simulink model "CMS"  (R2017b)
settings: Solver=FixedStepDiscrete  StartTime=0.0  StopTime=10.0  FixedStep=0.01  RelTol=1e-3  EnableMultiTasking=on
undefined symbols (not defined in the file): ASWTYPE_FALSE, ASWTYPE_TRUE, CcCMS_CANSendDelay_ms, CcCMS_ChrgMaxPackVoltLimt_V, CcCMS_PeakVoltCh_V, CcCMS_PeakVoltDisCh_V, CcSOC_DispSOCHighThrhd_pct, CMS09D_RUNTIME_MS, CMS_CONST0_NUMB, CMS_CONST1000_NUMB, CMS_CONST100_NUMB, CMS_CONST1_NUMB, CMS_CONST2047_NUMB, CMS_CONST2_NUMB, CMS_CONST3_NUMB, CMS_CONST4_NUMB, CMS_CONST5_NUMB, CMS_CONST6_NUMB, CMS_CONST7_NUMB, CMS_CONSTF1_NUMB, Enum_ACCACChrgState, Enum_CMSACChgMode, Enum_CMSBmsSelfChk, Enum_CMSBmsSt, Enum_CMSChgMode, Enum_CMSDCChgMode, Enum_CMSHVBatFltSevrtyStat, Enum_CMSHVConnSt, Enum_CMSPreThmMode, Enum_CMSPreThmReq, Enum_CMSThmPropagation, Enum_CTCCtrCtlConnMode, Enum_CTCCtrCtlState, Enum_DCCDCChrgState, Enum_DCCDCConnSt, Enum_ISOHVIsoFltLevel, Enum_MSMBMUState, Enum_ODPCCState, Enum_VDPPreThmEna
libraries: AIWAYS_Powertrain_BMS_lib x148
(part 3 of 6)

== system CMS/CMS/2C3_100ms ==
  GcCDP_MinCellVolt_mV : Inport
  GcCDP_MaxCellVolt_mV : Inport  Port=2
  GcBTM_CoolTempReq_C : Inport  Port=3
  GcBTM_HeatTempReq_C : Inport  Port=4
  GcCDP_MaxBusbarTemp_C : Inport  Port=5
  GcCDP_MinBusbarTemp_C : Inport  Port=6
  GcUDS_BusbarTempNumb_numb : Inport  Port=7
  GcCDP_MaxCellTemp_C : Inport  Port=8
  GcCDP_MinCellTemp_C : Inport  Port=9
  CMS_2C3_100ms : TriggerPort  TriggerType=function-call  VariantControl=(inherit)
  2C3_100ms_sys : Subsystem
  GcCMS_ClntTgtTemp_C : Outport
  GcCMS_HtTgtTemp_C : Outport  Port=2
  GcCMS_MaxCellVolt_V : Outport  Port=3
  GcCMS_BusbarTempMax_C : Outport  Port=4
  GcCMS_BusbarTempMin_C : Outport  Port=5
  GcCMS_MinCellVolt_V : Outport  Port=6
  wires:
  GcCDP_MinCellVolt_mV/1 -> 2C3_100ms_sys/1(GcCDP_MinCellVolt_mV)
  2C3_100ms_sys/1(GcCMS_ClntTgtTemp_C) -> GcCMS_ClntTgtTemp_C/1
  2C3_100ms_sys/2(GcCMS_HtTgtTemp_C) -> GcCMS_HtTgtTemp_C/1
  2C3_100ms_sys/3(GcCMS_MaxCellVolt_V) -> GcCMS_MaxCellVolt_V/1
  2C3_100ms_sys/4(GcCMS_BusbarTempMax_C) -> GcCMS_BusbarTempMax_C/1
  2C3_100ms_sys/5(GcCMS_BusbarTempMin_C) -> GcCMS_BusbarTempMin_C/1
  2C3_100ms_sys/6(GcCMS_MinCellVolt_V) -> GcCMS_MinCellVolt_V/1
  GcCDP_MaxCellVolt_mV/1 -> 2C3_100ms_sys/2(GcCDP_MaxCellVolt_mV)
  GcBTM_CoolTempReq_C/1 -> 2C3_100ms_sys/3(GcBTM_CoolTempReq_C)
  GcBTM_HeatTempReq_C/1 -> 2C3_100ms_sys/4(GcBTM_HeatTempReq_C)
  GcCDP_MaxBusbarTemp_C/1 -> 2C3_100ms_sys/5(GcCDP_MaxBusbarTemp_C)
  GcCDP_MinBusbarTemp_C/1 -> 2C3_100ms_sys/6(GcCDP_MinBusbarTemp_C)
  GcUDS_BusbarTempNumb_numb/1 -> 2C3_100ms_sys/7(GcUDS_BusbarTempNumb_numb)
  GcCDP_MaxCellTemp_C/1 -> 2C3_100ms_sys/8(GcCDP_MaxCellTemp_C)
  GcCDP_MinCellTemp_C/1 -> 2C3_100ms_sys/9(GcCDP_MinCellTemp_C)

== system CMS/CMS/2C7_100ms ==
  GbACC_ObcChrgCmd_flg : Inport
  GcHDP_PackVolt_V : Inport  Port=2
  GcHDP_PackCrnt_A : Inport  Port=3
  GcACC_ACChrgVoltRqst_V : Inport  Port=4
  GcACC_ACChrgCrntRqst_A : Inport  Port=5
  GbACC_ACChrgRqst_flg : Inport  Port=6
  GbODP_V2XDischrgCmd_flg : Inport  Port=7
  GbACC_PreThmObcChrgCmd_flg : Inport  Port=8
  GcACC_PreThmCrntRqst_A : Inport  Port=9
  GcACC_PreThmVoltRqst_V : Inport  Port=10
  GbACC_PreHeatPrmt_flg : Inport  Port=11
  GbACC_HoldTempObcChrgCmd_flg : Inport  Port=12
  GbACC_HoldTempPrmt_flg : Inport  Port=13
  GcACC_HoldTempVoltRqst_V : Inport  Port=14
  GcACC_HoldTempCrntRqst_A : Inport  Port=15
  CMS_2C7_100ms : TriggerPort  TriggerType=function-call  VariantControl=(inherit)
  2C7_100ms_sys : Subsystem
  GbCMS_ChrgCmd_flg : Outport
  GcCMS_ActPwrChrg_Kw : Outport  Port=2
  GcCMS_MaxVoltChrg_V : Outport  Port=3
  GcCMS_ReqVoltChrg_V : Outport  Port=4
  GcCMS_ReqCurrChrg_A : Outport  Port=5
  GbCMS_ObcRdyReq_flg : Outport  Port=6
  GbCMS_DischgCmd_flg : Outport  Port=7
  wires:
  GbACC_ObcChrgCmd_flg/1 -> 2C7_100ms_sys/1(GbACC_ObcChrgCmd_flg)
  GcHDP_PackVolt_V/1 -> 2C7_100ms_sys/2(GcHDP_PackVolt_V)
  GcHDP_PackCrnt_A/1 -> 2C7_100ms_sys/3(GcHDP_PackCrnt_A)
  GcACC_ACChrgVoltRqst_V/1 -> 2C7_100ms_sys/4(GcACC_ACChrgVoltRqst_V)
  GcACC_ACChrgCrntRqst_A/1 -> 2C7_100ms_sys/5(GcACC_ACChrgCrntRqst_A)
  GbACC_ACChrgRqst_flg/1 -> 2C7_100ms_sys/6(GbACC_ACChrgRqst_flg)
  2C7_100ms_sys/2(GcCMS_ActPwrChrg_Kw) -> GcCMS_ActPwrChrg_Kw/1
  2C7_100ms_sys/1(GbCMS_ChrgCmd_flg) -> GbCMS_ChrgCmd_flg/1
  2C7_100ms_sys/3(GcCMS_MaxVoltChrg_V) -> GcCMS_MaxVoltChrg_V/1
  2C7_100ms_sys/4(GcCMS_ReqVoltChrg_V) -> GcCMS_ReqVoltChrg_V/1
  2C7_100ms_sys/5(GcCMS_ReqCurrChrg_A) -> GcCMS_ReqCurrChrg_A/1
  2C7_100ms_sys/6(GbCMS_ObcRdyReq_flg) -> GbCMS_ObcRdyReq_flg/1
  2C7_100ms_sys/7(GbCMS_DischgCmd_flg) -> GbCMS_DischgCmd_flg/1
  GbODP_V2XDischrgCmd_flg/1 -> 2C7_100ms_sys/7(GbODP_V2XDischrgCmd_flg)
  GbACC_PreThmObcChrgCmd_flg/1 -> 2C7_100ms_sys/8(GbACC_PreThmObcChrgCmd_flg)
  GcACC_PreThmCrntRqst_A/1 -> 2C7_100ms_sys/9(GcACC_PreThmCrntRqst_A)
  GbACC_PreHeatPrmt_flg/1 -> 2C7_100ms_sys/10(GbACC_PreHeatPrmt_flg)
  GcACC_PreThmVoltRqst_V/1 -> 2C7_100ms_sys/11(GcACC_PreThmVoltRqst_V)
  GbACC_HoldTempObcChrgCmd_flg/1 -> 2C7_100ms_sys/12(GbACC_HoldTempObcChrgCmd_flg)
  GbACC_HoldTempPrmt_flg/1 -> 2C7_100ms_sys/13(GbACC_HoldTempPrmt_flg)
  GcACC_HoldTempVoltRqst_V/1 -> 2C7_100ms_sys/14(GcACC_HoldTempVoltRqst_V)
  GcACC_HoldTempCrntRqst_A/1 -> 2C7_100ms_sys/15(GcACC_HoldTempCrntRqst_A)

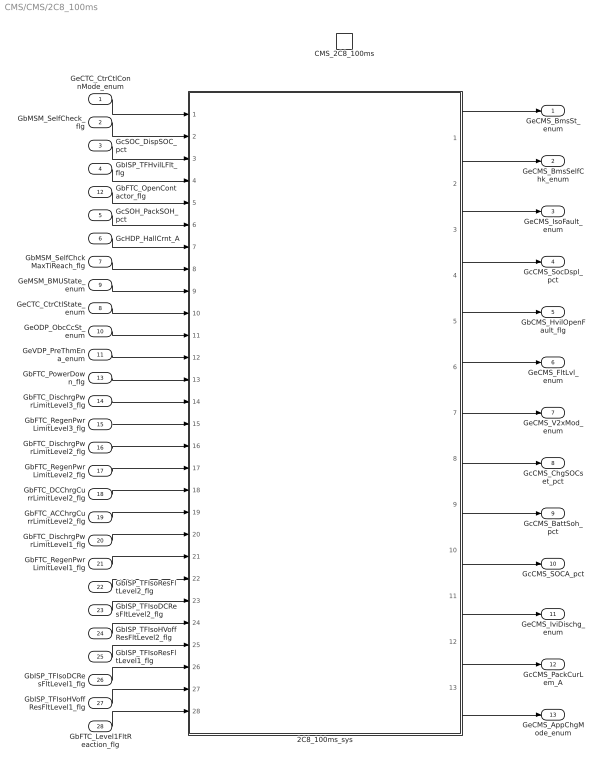
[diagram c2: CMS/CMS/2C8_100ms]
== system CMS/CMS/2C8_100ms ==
  GeCTC_CtrCtlConnMode_enum : Inport
  GbMSM_SelfCheck_flg : Inport  Port=2
  GcSOC_DispSOC_pct : Inport  Port=3
  GbISP_TFHvilLFlt_flg : Inport  Port=4
  GcSOH_PackSOH_pct : Inport  Port=5
  GcHDP_HallCrnt_A : Inport  Port=6
  GbMSM_SelfChckMaxTiReach_flg : Inport  Port=7
  GeCTC_CtrCtlState_enum : Inport  Port=8
  GeMSM_BMUState_enum : Inport  Port=9
  GeODP_ObcCcSt_enum : Inport  Port=10
  GeVDP_PreThmEna_enum : Inport  Port=11
  GbFTC_OpenContactor_flg : Inport  Port=12
  GbFTC_PowerDown_flg : Inport  Port=13
  GbFTC_DischrgPwrLimitLevel3_flg : Inport  Port=14
  GbFTC_RegenPwrLimitLevel3_flg : Inport  Port=15
  GbFTC_DischrgPwrLimitLevel2_flg : Inport  Port=16
  GbFTC_RegenPwrLimitLevel2_flg : Inport  Port=17
  GbFTC_DCChrgCurrLimitLevel2_flg : Inport  Port=18
  GbFTC_ACChrgCurrLimitLevel2_flg : Inport  Port=19
  GbFTC_DischrgPwrLimitLevel1_flg : Inport  Port=20
  GbFTC_RegenPwrLimitLevel1_flg : Inport  Port=21
  GbISP_TFIsoResFltLevel2_flg : Inport  Port=22
  GbISP_TFIsoDCResFltLevel2_flg : Inport  Port=23
  GbISP_TFIsoHVoffResFltLevel2_flg : Inport  Port=24
  GbISP_TFIsoResFltLevel1_flg : Inport  Port=25
  GbISP_TFIsoDCResFltLevel1_flg : Inport  Port=26
  GbISP_TFIsoHVoffResFltLevel1_flg : Inport  Port=27
  GbFTC_Level1FltReaction_flg : Inport  Port=28
  CMS_2C8_100ms : TriggerPort  TriggerType=function-call  VariantControl=(inherit)
  2C8_100ms_sys : Subsystem
  GeCMS_BmsSt_enum : Outport
  GeCMS_BmsSelfChk_enum : Outport  Port=2
  GeCMS_IsoFault_enum : Outport  Port=3
  GcCMS_SocDspl_pct : Outport  Port=4
  GbCMS_HvilOpenFault_flg : Outport  Port=5
  GeCMS_FltLvl_enum : Outport  Port=6
  GeCMS_V2xMod_enum : Outport  Port=7
  GcCMS_ChgSOCset_pct : Outport  Port=8
  GcCMS_BattSoh_pct : Outport  Port=9
  GcCMS_SOCA_pct : Outport  Port=10
  GeCMS_IviDischg_enum : Outport  Port=11
  GcCMS_PackCurLem_A : Outport  Port=12
  GeCMS_AppChgMode_enum : Outport  Port=13
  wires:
  GeCTC_CtrCtlConnMode_enum/1 -> 2C8_100ms_sys/1(GeCTC_CtrCtlConnMode_enum)
  GbMSM_SelfCheck_flg/1 -> 2C8_100ms_sys/2(GbMSM_SelfCheck_flg)
  GcSOC_DispSOC_pct/1 -> 2C8_100ms_sys/3(GcSOC_DispSOC_pct)
  GbISP_TFHvilLFlt_flg/1 -> 2C8_100ms_sys/4(GbISP_TFHvilLFlt_flg)
  GbFTC_OpenContactor_flg/1 -> 2C8_100ms_sys/5(GbFTC_OpenContactor_flg)
  GcSOH_PackSOH_pct/1 -> 2C8_100ms_sys/6(GcSOH_PackSOH_pct)
  GcHDP_HallCrnt_A/1 -> 2C8_100ms_sys/7(GcHDP_HallCrnt_A)
  2C8_100ms_sys/1(GeCMS_BmsSt_enum) -> GeCMS_BmsSt_enum/1
  2C8_100ms_sys/2(GeCMS_BmsSelfChk_enum) -> GeCMS_BmsSelfChk_enum/1
  2C8_100ms_sys/3(GeCMS_IsoFault_enum) -> GeCMS_IsoFault_enum/1
  2C8_100ms_sys/4(GcCMS_SocDspl_pct) -> GcCMS_SocDspl_pct/1
  2C8_100ms_sys/5(GbCMS_HvilOpenFault_flg) -> GbCMS_HvilOpenFault_flg/1
  2C8_100ms_sys/6(GeCMS_FltLvl_enum) -> GeCMS_FltLvl_enum/1
  2C8_100ms_sys/7(GeCMS_V2xMod_enum) -> GeCMS_V2xMod_enum/1
  2C8_100ms_sys/8(GcCMS_ChgSOCset_pct) -> GcCMS_ChgSOCset_pct/1
  2C8_100ms_sys/9(GcCMS_BattSoh_pct) -> GcCMS_BattSoh_pct/1
  2C8_100ms_sys/10(GcCMS_SOCA_pct) -> GcCMS_SOCA_pct/1
  2C8_100ms_sys/11(GeCMS_IviDischg_enum) -> GeCMS_IviDischg_enum/1
  2C8_100ms_sys/12(GcCMS_PackCurLem_A) -> GcCMS_PackCurLem_A/1
  GbMSM_SelfChckMaxTiReach_flg/1 -> 2C8_100ms_sys/8(GbMSM_SelfChckMaxTiReach_flg)
  GeCTC_CtrCtlState_enum/1 -> 2C8_100ms_sys/10(GeCTC_CtrCtlState_enum)
  GeMSM_BMUState_enum/1 -> 2C8_100ms_sys/9(GeMSM_BMUState_enum)
  GeODP_ObcCcSt_enum/1 -> 2C8_100ms_sys/11(GeODP_ObcCcSt_enum)
  GeVDP_PreThmEna_enum/1 -> 2C8_100ms_sys/12(GeVDP_PreThmEna_enum)
  GbFTC_PowerDown_flg/1 -> 2C8_100ms_sys/13(GbFTC_PowerDown_flg)
  GbFTC_DischrgPwrLimitLevel3_flg/1 -> 2C8_100ms_sys/14(GbFTC_DischrgPwrLimitLevel3_flg)
  GbFTC_RegenPwrLimitLevel3_flg/1 -> 2C8_100ms_sys/15(GbFTC_RegenPwrLimitLevel3_flg)
  GbFTC_DischrgPwrLimitLevel2_flg/1 -> 2C8_100ms_sys/16(GbFTC_DischrgPwrLimitLevel2_flg)
  GbFTC_RegenPwrLimitLevel2_flg/1 -> 2C8_100ms_sys/17(GbFTC_RegenPwrLimitLevel2_flg)
  GbFTC_DCChrgCurrLimitLevel2_flg/1 -> 2C8_100ms_sys/18(GbFTC_DCChrgCurrLimitLevel2_flg)
  GbFTC_ACChrgCurrLimitLevel2_flg/1 -> 2C8_100ms_sys/19(GbFTC_ACChrgCurrLimitLevel2_flg)
  GbFTC_DischrgPwrLimitLevel1_flg/1 -> 2C8_100ms_sys/20(GbFTC_DischrgPwrLimitLevel1_flg)
  GbFTC_RegenPwrLimitLevel1_flg/1 -> 2C8_100ms_sys/21(GbFTC_RegenPwrLimitLevel1_flg)
  2C8_100ms_sys/13(GeCMS_AppChgMode_enum) -> GeCMS_AppChgMode_enum/1
  GbISP_TFIsoResFltLevel2_flg/1 -> 2C8_100ms_sys/22(GbISP_TFIsoResFltLevel2_flg)
  GbISP_TFIsoDCResFltLevel2_flg/1 -> 2C8_100ms_sys/23(GbISP_TFIsoDCResFltLevel2_flg)
  GbISP_TFIsoHVoffResFltLevel2_flg/1 -> 2C8_100ms_sys/24(GbISP_TFIsoHVoffResFltLevel2_flg)
  GbISP_TFIsoResFltLevel1_flg/1 -> 2C8_100ms_sys/25(GbISP_TFIsoResFltLevel1_flg)
  GbISP_TFIsoDCResFltLevel1_flg/1 -> 2C8_100ms_sys/26(GbISP_TFIsoDCResFltLevel1_flg)
  GbISP_TFIsoHVoffResFltLevel1_flg/1 -> 2C8_100ms_sys/27(GbISP_TFIsoHVoffResFltLevel1_flg)
  GbFTC_Level1FltReaction_flg/1 -> 2C8_100ms_sys/28(GbFTC_Level1FltReaction_flg)

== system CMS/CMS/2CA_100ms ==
  GaCDP_CellBalc_flg : Inport
  GbDCC_DCChrgRqst_flg : Inport  Port=2
  GbACC_ACChrgRqst_flg : Inport  Port=3
  GeCTC_CtrCtlConnMode_enum : Inport  Port=4
  GbADP_DischgReq_flg : Inport  Port=5
  GcHDP_PackVolt_V : Inport  Port=6
  GbACC_PreThmRqst_flg : Inport  Port=7
  GbFTC_PowerDown_flg : Inport  Port=8
  GbACC_PreHeatPrmt_flg : Inport  Port=9
  GeVDP_PreThmEna_enum : Inport  Port=10
  GcSOP_DischrgConstPwr_kW : Inport  Port=11
  GcSOP_ChrgConstPwr_kW : Inport  Port=12
  GbACC_HoldTempPrmt_flg : Inport  Port=13
  GbACC_HoldTempRqst_flg : Inport  Port=14
  CMS_2CA_100ms : TriggerPort  TriggerType=function-call  VariantControl=(inherit)
  2CA_100ms_sys : Subsystem
  GcCMS_BattInVolt_V : Outport
  GbCMS_BalSt_flg : Outport  Port=2
  GbCMS_BalVlg_flg : Outport  Port=3
  GbCMS_VcuPwrUpReq_flg : Outport  Port=4
  GbCMS_VcuPwrUpReqVld_flg : Outport  Port=5
  GcCMS_ConstCurrDisChMax_A : Outport  Port=6
  GcCMS_ConstCurrChMax_A : Outport  Port=7
  GbCMS_PwrDownReq_flg : Outport  Port=8
  GbCMS_PwrDownReqVld_flg : Outport  Port=9
  GeCMS_ChrgPreThmMode_enum : Outport  Port=10
  GeCMS_ElockReq_enum : Outport  Port=11
  GeCMS_PreThmReq_enum : Outport  Port=12
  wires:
  2CA_100ms_sys/1(GcCMS_BattInVolt_V) -> GcCMS_BattInVolt_V/1
  2CA_100ms_sys/2(GbCMS_BalSt_flg) -> GbCMS_BalSt_flg/1
  2CA_100ms_sys/3(GbCMS_BalVlg_flg) -> GbCMS_BalVlg_flg/1
  2CA_100ms_sys/4(GbCMS_VcuPwrUpReq_flg) -> GbCMS_VcuPwrUpReq_flg/1
  2CA_100ms_sys/5(GbCMS_VcuPwrUpReqVld_flg) -> GbCMS_VcuPwrUpReqVld_flg/1
  2CA_100ms_sys/6(GcCMS_ConstCurrDisChMax_A) -> GcCMS_ConstCurrDisChMax_A/1
  2CA_100ms_sys/7(GcCMS_ConstCurrChMax_A) -> GcCMS_ConstCurrChMax_A/1
  2CA_100ms_sys/8(GbCMS_PwrDownReq_flg) -> GbCMS_PwrDownReq_flg/1
  2CA_100ms_sys/9(GbCMS_PwrDownReqVld_flg) -> GbCMS_PwrDownReqVld_flg/1
  2CA_100ms_sys/10(GeCMS_ChrgPreThmMode_enum) -> GeCMS_ChrgPreThmMode_enum/1
  2CA_100ms_sys/11(GeCMS_ElockReq_enum) -> GeCMS_ElockReq_enum/1
  2CA_100ms_sys/12(GeCMS_PreThmReq_enum) -> GeCMS_PreThmReq_enum/1
  GeCTC_CtrCtlConnMode_enum/1 -> 2CA_100ms_sys/4(GeCTC_CtrCtlConnMode_enum)
  GbACC_ACChrgRqst_flg/1 -> 2CA_100ms_sys/3(GbACC_ACChrgRqst_flg)
  GbDCC_DCChrgRqst_flg/1 -> 2CA_100ms_sys/2(GbDCC_DCChrgRqst_flg)
  GaCDP_CellBalc_flg/1 -> 2CA_100ms_sys/1(GaCDP_CellBalc_flg)
  GbADP_DischgReq_flg/1 -> 2CA_100ms_sys/5(GbADP_DischgReq_flg)
  GcHDP_PackVolt_V/1 -> 2CA_100ms_sys/6(GcHDP_PackVolt_V)
  GbACC_PreThmRqst_flg/1 -> 2CA_100ms_sys/7(GbACC_PreThmRqst_flg)
  GbFTC_PowerDown_flg/1 -> 2CA_100ms_sys/8(GbFTC_PowerDown_flg)
  GbACC_PreHeatPrmt_flg/1 -> 2CA_100ms_sys/9(GbACC_PreHeatPrmt_flg)
  GeVDP_PreThmEna_enum/1 -> 2CA_100ms_sys/10(GeVDP_PreThmEna_enum)
  GcSOP_DischrgConstPwr_kW/1 -> 2CA_100ms_sys/11(GcSOP_DischrgConstPwr_kW)
  GcSOP_ChrgConstPwr_kW/1 -> 2CA_100ms_sys/12(GcSOP_ChrgConstPwr_kW)
  GbACC_HoldTempPrmt_flg/1 -> 2CA_100ms_sys/13(GbACC_HoldTempPrmt_flg)
  GbACC_HoldTempRqst_flg/1 -> 2CA_100ms_sys/14(GbACC_HoldTempRqst_flg)

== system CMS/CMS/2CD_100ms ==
  GcSOP_DischrgPwr_kW : Inport
  GcSOP_ChrgPwr_kW : Inport  Port=2
  GcSOP_DischrgConstPwr_kW : Inport  Port=3
  GcSOP_ChrgConstPwr_kW : Inport  Port=4
  CMS_2CD_100ms : TriggerPort  TriggerType=function-call  VariantControl=(inherit)
  2CD_100ms_sys : Subsystem
  GcCMS_PeakPwrDisCh_Kw : Outport
  GcCMS_PeakPwrCh_Kw : Outport  Port=2
  GcCMS_ConstPwrDisCh_Kw : Outport  Port=3
  GcCMS_ConstPwrCh_Kw : Outport  Port=4
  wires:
  GcSOP_DischrgConstPwr_kW/1 -> 2CD_100ms_sys/3(GcSOP_DischrgConstPwr_kW)
  GcSOP_ChrgConstPwr_kW/1 -> 2CD_100ms_sys/4(GcSOP_ChrgConstPwr_kW)
  2CD_100ms_sys/1(GcCMS_PeakPwrDisCh_Kw) -> GcCMS_PeakPwrDisCh_Kw/1
  2CD_100ms_sys/2(GcCMS_PeakPwrCh_Kw) -> GcCMS_PeakPwrCh_Kw/1
  2CD_100ms_sys/3(GcCMS_ConstPwrDisCh_Kw) -> GcCMS_ConstPwrDisCh_Kw/1
  2CD_100ms_sys/4(GcCMS_ConstPwrCh_Kw) -> GcCMS_ConstPwrCh_Kw/1
  GcSOP_DischrgPwr_kW/1 -> 2CD_100ms_sys/1(GcSOP_DischrgPwr_kW)
  GcSOP_ChrgPwr_kW/1 -> 2CD_100ms_sys/2(GcSOP_ChrgPwr_kW)

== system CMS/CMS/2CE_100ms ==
  GcISO_HVIsoValue_kohm : Inport
  GeODP_ObcCcSt_enum : Inport  Port=2
  GbDCC_DCChrgFinish_flg : Inport  Port=3
  GbACC_ACChrgFinish_flg : Inport  Port=4
  GcSOC_PackSOC_pct : Inport  Port=5
  GeACC_ACChrgState_enum : Inport  Port=6
  GeDCC_DCConnSt_enum : Inport  Port=7
  GeLDP_CC2St_enum : Inport  Port=8
  GcACC_ChrgingTiRem_min : Inport  Port=9
  GcDCC_ChrgingTiRem_min : Inport  Port=10
  GeCTC_CtrCtlConnMode_enum : Inport  Port=11
  GbACC_PreHeatPrmt_flg : Inport  Port=12
  GeVDP_PreThmEna_enum : Inport  Port=13
  GeDCC_DCChrgState_enum : Inport  Port=14
  GeLDP_ChrgGunConnSt_enum : Inport  Port=15
  CMS_2CE_100ms : TriggerPort  TriggerType=function-call  VariantControl=(inherit)
  2CE_100ms_sys : Subsystem
  GcCMS_ResIso_Kohm : Outport
  GcCMS_ChrgRemTime_Min : Outport  Port=2
  GeCMS_ACPlugCnnt_enum : Outport  Port=3
  GbCMS_BattFull_flg : Outport  Port=4
  GbCMS_WarnLamp_flg : Outport  Port=5
  GbCMS_SerLamp_flg : Outport  Port=6
  GbCMS_TempDiffWarn_flg : Outport  Port=7
  GbCMS_OverChrgWarn_flg : Outport  Port=8
  GbCMS_ConsisWarn_flg : Outport  Port=9
  GbCMS_MishWarn_flg : Outport  Port=10
  GbCMS_SocHopWarn_flg : Outport  Port=11
  GbCMS_SocHighWarn_flg : Outport  Port=12
  GbCMS_SocLowWarn_flg : Outport  Port=13
  GbCMS_OTAModeSt_flg : Outport  Port=14
  GeCMS_AcDcConnBoth_enum : Outport  Port=15
  GbCMS_CellUvFlt_flg : Outport  Port=16
  GbCMS_CellOvFlt_flg : Outport  Port=17
  GbCMS_PackUvFlt_flg : Outport  Port=18
  GbCMS_PackOvFlt_flg : Outport  Port=19
  GbCMS_TempHighWarn_flg : Outport  Port=20
  GcCMS_RealSoc_pct : Outport  Port=21
  GeCMS_DCPlugConn_enum : Outport  Port=22
  GeCMS_ACChgMode_enum : Outport  Port=23
  GeCMS_DCChgMode_enum : Outport  Port=24
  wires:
  GeODP_ObcCcSt_enum/1 -> 2CE_100ms_sys/2(GeODP_ObcCcSt_enum)
  GcISO_HVIsoValue_kohm/1 -> 2CE_100ms_sys/1(GcISO_HVIsoValue_kohm)
  GbDCC_DCChrgFinish_flg/1 -> 2CE_100ms_sys/3(GbDCC_DCChrgFinish_flg)
  GbACC_ACChrgFinish_flg/1 -> 2CE_100ms_sys/4(GbACC_ACChrgFinish_flg)
  GcSOC_PackSOC_pct/1 -> 2CE_100ms_sys/5(GcSOC_PackSOC_pct)
  2CE_100ms_sys/1(GcCMS_ResIso_Kohm) -> GcCMS_ResIso_Kohm/1
  2CE_100ms_sys/2(GcCMS_ChrgRemTime_Min) -> GcCMS_ChrgRemTime_Min/1
  2CE_100ms_sys/3(GeCMS_ACPlugCnnt_enum) -> GeCMS_ACPlugCnnt_enum/1
  2CE_100ms_sys/4(GbCMS_BattFull_flg) -> GbCMS_BattFull_flg/1
  2CE_100ms_sys/5(GbCMS_WarnLamp_flg) -> GbCMS_WarnLamp_flg/1
  2CE_100ms_sys/6(GbCMS_SerLamp_flg) -> GbCMS_SerLamp_flg/1
  2CE_100ms_sys/7(GbCMS_TempDiffWarn_flg) -> GbCMS_TempDiffWarn_flg/1
  2CE_100ms_sys/8(GbCMS_OverChrgWarn_flg) -> GbCMS_OverChrgWarn_flg/1
  2CE_100ms_sys/9(GbCMS_ConsisWarn_flg) -> GbCMS_ConsisWarn_flg/1
  2CE_100ms_sys/10(GbCMS_MishWarn_flg) -> GbCMS_MishWarn_flg/1
  2CE_100ms_sys/11(GbCMS_SocHopWarn_flg) -> GbCMS_SocHopWarn_flg/1
  2CE_100ms_sys/12(GbCMS_SocHighWarn_flg) -> GbCMS_SocHighWarn_flg/1
  2CE_100ms_sys/13(GbCMS_SocLowWarn_flg) -> GbCMS_SocLowWarn_flg/1
  2CE_100ms_sys/14(GbCMS_OTAModeSt_flg) -> GbCMS_OTAModeSt_flg/1
  2CE_100ms_sys/15(GeCMS_AcDcConnBoth_enum) -> GeCMS_AcDcConnBoth_enum/1
  2CE_100ms_sys/16(GbCMS_CellUvFlt_flg) -> GbCMS_CellUvFlt_flg/1
  2CE_100ms_sys/17(GbCMS_CellOvFlt_flg) -> GbCMS_CellOvFlt_flg/1
  2CE_100ms_sys/18(GbCMS_PackUvFlt_flg) -> GbCMS_PackUvFlt_flg/1
  2CE_100ms_sys/19(GbCMS_PackOvFlt_flg) -> GbCMS_PackOvFlt_flg/1
  2CE_100ms_sys/20(GbCMS_TempHighWarn_flg) -> GbCMS_TempHighWarn_flg/1
  2CE_100ms_sys/21(GcCMS_RealSoc_pct) -> GcCMS_RealSoc_pct/1
  2CE_100ms_sys/22(GeCMS_DCPlugConn_enum) -> GeCMS_DCPlugConn_enum/1
  2CE_100ms_sys/23(GeCMS_ACChgMode_enum) -> GeCMS_ACChgMode_enum/1
  2CE_100ms_sys/24(GeCMS_DCChgMode_enum) -> GeCMS_DCChgMode_enum/1
  GeACC_ACChrgState_enum/1 -> 2CE_100ms_sys/6(GeACC_ACChrgState_enum)
  GeDCC_DCConnSt_enum/1 -> 2CE_100ms_sys/7(GeDCC_DCConnSt_enum)
  GeLDP_CC2St_enum/1 -> 2CE_100ms_sys/8(GeLDP_CC2St_enum)
  GcACC_ChrgingTiRem_min/1 -> 2CE_100ms_sys/9(GcACC_ChrgingTiRem_min)
  GcDCC_ChrgingTiRem_min/1 -> 2CE_100ms_sys/10(GcDCC_ChrgingTiRem_min)
  GeCTC_CtrCtlConnMode_enum/1 -> 2CE_100ms_sys/11(GeCTC_CtrCtlConnMode_enum)
  GbACC_PreHeatPrmt_flg/1 -> 2CE_100ms_sys/12(GbACC_PreHeatPrmt_flg)
  GeVDP_PreThmEna_enum/1 -> 2CE_100ms_sys/13(GeVDP_PreThmEna_enum)
  GeDCC_DCChrgState_enum/1 -> 2CE_100ms_sys/14(GeDCC_DCChrgState_enum)
  GeLDP_ChrgGunConnSt_enum/1 -> 2CE_100ms_sys/15(GeLDP_ChrgGunConnSt_enum)

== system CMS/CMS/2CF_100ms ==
  GcCDP_AvgCellTemp_C : Inport
  GbISO_IsoForbid_flg : Inport  Port=2
  GcCDP_MaxCellTemp_C : Inport  Port=3
  GcCDP_MinCellTemp_C : Inport  Port=4
  GcSOC_DispSOC_pct : Inport  Port=5
  GcHDP_FuseVolt_V : Inport  Port=6
  GcUDS_BatEnergy_kWh : Inport  Port=7
  GcUDS_CellTempNumb_numb : Inport  Port=8
  GcCDP_MaxBusbarTemp_C : Inport  Port=9
  GcCDP_MinBusbarTemp_C : Inport  Port=10
  CMS_2CF_100ms : TriggerPort  TriggerType=function-call  VariantControl=(inherit)
  2CF_100ms_sys : Subsystem
  GcCMS_BattTempAvrg_C : Outport
  GcCMS_BattNrmEnrg_kwh : Outport  Port=2
  GbCMS_BattTempFault_flg : Outport  Port=3
  GcCMS_BattSoe_kwh : Outport  Port=4
  GbCMS_IsoChkSt_flg : Outport  Port=5
  GcCMS_BattTempMax_C : Outport  Port=6
  GcCMS_BattTempMin_C : Outport  Port=7
  GcCMS_FuseVolt_V : Outport  Port=8
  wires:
  GbISO_IsoForbid_flg/1 -> 2CF_100ms_sys/2(GbISO_IsoForbid_flg)
  GcCDP_AvgCellTemp_C/1 -> 2CF_100ms_sys/1(GcCDP_AvgCellTemp_C)
  GcCDP_MaxCellTemp_C/1 -> 2CF_100ms_sys/3(GcCDP_MaxCellTemp_C)
  GcCDP_MinCellTemp_C/1 -> 2CF_100ms_sys/4(GcCDP_MinCellTemp_C)
  2CF_100ms_sys/1(GcCMS_BattTempAvrg_C) -> GcCMS_BattTempAvrg_C/1
  2CF_100ms_sys/2(GcCMS_BattNrmEnrg_kwh) -> GcCMS_BattNrmEnrg_kwh/1
  2CF_100ms_sys/3(GbCMS_BattTempFault_flg) -> GbCMS_BattTempFault_flg/1
  2CF_100ms_sys/4(GcCMS_BattSoe_kwh) -> GcCMS_BattSoe_kwh/1
  2CF_100ms_sys/5(GbCMS_IsoChkSt_flg) -> GbCMS_IsoChkSt_flg/1
  2CF_100ms_sys/6(GcCMS_BattTempMax_C) -> GcCMS_BattTempMax_C/1
  2CF_100ms_sys/7(GcCMS_BattTempMin_C) -> GcCMS_BattTempMin_C/1
  2CF_100ms_sys/8(GcCMS_FuseVolt_V) -> GcCMS_FuseVolt_V/1
  GcSOC_DispSOC_pct/1 -> 2CF_100ms_sys/5(GcSOC_DispSOC_pct)
  GcHDP_FuseVolt_V/1 -> 2CF_100ms_sys/6(GcHDP_FuseVolt_V)
  GcUDS_BatEnergy_kWh/1 -> 2CF_100ms_sys/7(GcUDS_BatEnergy_kWh)
  GcUDS_CellTempNumb_numb/1 -> 2CF_100ms_sys/8(GcUDS_CellTempNumb_numb)
  GcCDP_MaxBusbarTemp_C/1 -> 2CF_100ms_sys/9(GcCDP_MaxBusbarTemp_C)
  GcCDP_MinBusbarTemp_C/1 -> 2CF_100ms_sys/10(GcCDP_MinBusbarTemp_C)

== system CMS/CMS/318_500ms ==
  GcCDP_MaxCellVoltNumb_numb : Inport
  GcCDP_MinCellVoltNumb_numb : Inport  Port=2
  GcCDP_MaxCellTempNumb_numb : Inport  Port=3
  GcCDP_MinCellTempNumb_numb : Inport  Port=4
  GbWSM_DCWkUpPrs_flg : Inport  Port=5
  GeCMS_ACChgMode_enum : Inport  Port=6
  GeCMS_DCChgMode_enum : Inport  Port=7
  CMS_318_500ms : TriggerPort  TriggerType=function-call  VariantControl=(inherit)
  318_500ms_sys : Subsystem
  GcCMS_MaxCellVoltNumb_numb : Outport
  GcCMS_MinCellVoltNumb_numb : Outport  Port=2
  GcCMS_MaxCellTempNumb_numb : Outport  Port=3
  GcCMS_MinCellTempNumb_numb : Outport  Port=4
  GcCMS_MaxVoltNumb_numb : Outport  Port=5
  GcCMS_MinVoltNumb_numb : Outport  Port=6
  GcCMS_MaxTempNumb_numb : Outport  Port=7
  GcCMS_MinTempNumb_numb : Outport  Port=8
  GeCMS_ChgMode_enum : Outport  Port=9
  GeCMS_DChrgModeDebug_enum : Outport  Port=10
  GbCMS_DChrgWkUp_flg : Outport  Port=11
  GeCMS_EvccMode_enum : Outport  Port=12
  GeCMS_AChrgObsr_enum : Outport  Port=13
  GeCMS_PreThmObsvr_enum : Outport  Port=14
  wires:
  GcCDP_MaxCellVoltNumb_numb/1 -> 318_500ms_sys/1(GcCDP_MaxCellVoltNumb_numb)
  GcCDP_MinCellTempNumb_numb/1 -> 318_500ms_sys/4(GcCDP_MinCellTempNumb_numb)
  GcCDP_MaxCellTempNumb_numb/1 -> 318_500ms_sys/3(GcCDP_MaxCellTempNumb_numb)
  GcCDP_MinCellVoltNumb_numb/1 -> 318_500ms_sys/2(GcCDP_MinCellVoltNumb_numb)
  GbWSM_DCWkUpPrs_flg/1 -> 318_500ms_sys/5(GbWSM_DCWkUpPrs_flg)
  318_500ms_sys/1(GcCMS_MaxCellVoltNumb_numb) -> GcCMS_MaxCellVoltNumb_numb/1
  318_500ms_sys/2(GcCMS_MinCellVoltNumb_numb) -> GcCMS_MinCellVoltNumb_numb/1
  318_500ms_sys/3(GcCMS_MaxCellTempNumb_numb) -> GcCMS_MaxCellTempNumb_numb/1
  318_500ms_sys/4(GcCMS_MinCellTempNumb_numb) -> GcCMS_MinCellTempNumb_numb/1
  318_500ms_sys/6(GcCMS_MinVoltNumb_numb) -> GcCMS_MinVoltNumb_numb/1
  318_500ms_sys/5(GcCMS_MaxVoltNumb_numb) -> GcCMS_MaxVoltNumb_numb/1
  318_500ms_sys/7(GcCMS_MaxTempNumb_numb) -> GcCMS_MaxTempNumb_numb/1
  318_500ms_sys/8(GcCMS_MinTempNumb_numb) -> GcCMS_MinTempNumb_numb/1
  318_500ms_sys/9(GeCMS_ChgMode_enum) -> GeCMS_ChgMode_enum/1
  318_500ms_sys/10(GeCMS_DChrgModeDebug_enum) -> GeCMS_DChrgModeDebug_enum/1
  318_500ms_sys/11(GbCMS_DChrgWkUp_flg) -> GbCMS_DChrgWkUp_flg/1
  318_500ms_sys/12(GeCMS_EvccMode_enum) -> GeCMS_EvccMode_enum/1
  318_500ms_sys/13(GeCMS_AChrgObsr_enum) -> GeCMS_AChrgObsr_enum/1
  318_500ms_sys/14(GeCMS_PreThmObsvr_enum) -> GeCMS_PreThmObsvr_enum/1
  GeCMS_ACChgMode_enum/1 -> 318_500ms_sys/6(GeCMS_ACChgMode_enum)
  GeCMS_DCChgMode_enum/1 -> 318_500ms_sys/7(GeCMS_DCChgMode_enum)

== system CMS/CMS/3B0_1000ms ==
  GcDCS_3072ChrgVoltReq_V : Inport
  GcDCC_DCChrgCrntRqst_A : Inport  Port=2
  CMS_3B0_1000ms : TriggerPort  TriggerType=function-call  VariantControl=(inherit)
  3B0_1000ms_sys : Subsystem
  GcCMS_ChrgAccum_Ah : Outport
  GbCMS_DChgStVoltOut_flg : Outport  Port=2
  GcCMS_DChrgVoltReq_V : Outport  Port=3
  GcCMS_DChrgCurrReq_A : Outport  Port=4
  GcCMS_DChrgRchSocLmt_numb : Outport  Port=5
  GcCMS_DChrgRchPackVoltLmt_numb : Outport  Port=6
  GcCMS_DChrgRchCellVoltLmt_numb : Outport  Port=7
  GcCMS_DChrgChrgerActStop_numb : Outport  Port=8
  GcCMS_DChrgBattInsulationErr_numb : Outport  Port=9
  GcCMS_DChrgOutpCnntOvrTempErr_numb : Outport  Port=10
  GcCMS_PcbOvrTempErr_numb : Outport  Port=11
  GcCMS_ChrgCnntErr_numb : Outport  Port=12
  GcCMS_BattOvrTempErr_numb : Outport  Port=13
  GcCMS_MainRelayErr_numb : Outport  Port=14
  GcCMS_CC2ChkVoltErr_numb : Outport  Port=15
  GcCMS_OtherErr_numb : Outport  Port=16
  GcCMS_ChrgCurrAbnrm_numb : Outport  Port=17
  GcCMS_ChrgVoltAbnrm_numb : Outport  Port=18
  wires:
  GcDCS_3072ChrgVoltReq_V/1 -> 3B0_1000ms_sys/1(GcDCS_3072ChrgVoltReq_V)
  GcDCC_DCChrgCrntRqst_A/1 -> 3B0_1000ms_sys/2(GcDCC_DCChrgCrntRqst_A)
  3B0_1000ms_sys/1(GcCMS_ChrgAccum_Ah) -> GcCMS_ChrgAccum_Ah/1
  3B0_1000ms_sys/2(GbCMS_DChgStVoltOut_flg) -> GbCMS_DChgStVoltOut_flg/1
  3B0_1000ms_sys/3(GcCMS_DChrgVoltReq_V) -> GcCMS_DChrgVoltReq_V/1
  3B0_1000ms_sys/4(GcCMS_DChrgCurrReq_A) -> GcCMS_DChrgCurrReq_A/1
  3B0_1000ms_sys/5(GcCMS_DChrgRchSocLmt_numb) -> GcCMS_DChrgRchSocLmt_numb/1
  3B0_1000ms_sys/6(GcCMS_DChrgRchPackVoltLmt_numb) -> GcCMS_DChrgRchPackVoltLmt_numb/1
  3B0_1000ms_sys/7(GcCMS_DChrgRchCellVoltLmt_numb) -> GcCMS_DChrgRchCellVoltLmt_numb/1
  3B0_1000ms_sys/8(GcCMS_DChrgChrgerActStop_numb) -> GcCMS_DChrgChrgerActStop_numb/1
  3B0_1000ms_sys/9(GcCMS_DChrgBattInsulationErr_numb) -> GcCMS_DChrgBattInsulationErr_numb/1
  3B0_1000ms_sys/10(GcCMS_DChrgOutpCnntOvrTempErr_numb) -> GcCMS_DChrgOutpCnntOvrTempErr_numb/1
  3B0_1000ms_sys/11(GcCMS_PcbOvrTempErr_numb) -> GcCMS_PcbOvrTempErr_numb/1
  3B0_1000ms_sys/12(GcCMS_ChrgCnntErr_numb) -> GcCMS_ChrgCnntErr_numb/1
  3B0_1000ms_sys/13(GcCMS_BattOvrTempErr_numb) -> GcCMS_BattOvrTempErr_numb/1
  3B0_1000ms_sys/14(GcCMS_MainRelayErr_numb) -> GcCMS_MainRelayErr_numb/1
  3B0_1000ms_sys/15(GcCMS_CC2ChkVoltErr_numb) -> GcCMS_CC2ChkVoltErr_numb/1
  3B0_1000ms_sys/16(GcCMS_OtherErr_numb) -> GcCMS_OtherErr_numb/1
  3B0_1000ms_sys/17(GcCMS_ChrgCurrAbnrm_numb) -> GcCMS_ChrgCurrAbnrm_numb/1
  3B0_1000ms_sys/18(GcCMS_ChrgVoltAbnrm_numb) -> GcCMS_ChrgVoltAbnrm_numb/1

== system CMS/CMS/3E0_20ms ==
  GaCDP_CellVolt_mV : Inport
  GcUDS_CellVoltNum_numb : Inport  Port=2
  CMS_3E0_20ms : TriggerPort  TriggerType=function-call  VariantControl=(inherit)
  3E0_20ms_sys : Subsystem
  GcCMS_CellVoltCnt_numb : Outport
  GcCMS_CellVolt1_V : Outport  Port=2
  GcCMS_CellVolt2_V : Outport  Port=3
  GcCMS_CellVolt3_V : Outport  Port=4
  GcCMS_CellVolt4_V : Outport  Port=5
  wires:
  3E0_20ms_sys/1(GcCMS_CellVoltCnt_numb) -> GcCMS_CellVoltCnt_numb/1
  3E0_20ms_sys/2(GcCMS_CellVolt1_V) -> GcCMS_CellVolt1_V/1
  3E0_20ms_sys/3(GcCMS_CellVolt2_V) -> GcCMS_CellVolt2_V/1
  3E0_20ms_sys/4(GcCMS_CellVolt3_V) -> GcCMS_CellVolt3_V/1
  3E0_20ms_sys/5(GcCMS_CellVolt4_V) -> GcCMS_CellVolt4_V/1
  GaCDP_CellVolt_mV/1 -> 3E0_20ms_sys/1(GaCDP_CellVolt_mV)
  GcUDS_CellVoltNum_numb/1 -> 3E0_20ms_sys/2(GcUDS_CellVoltNum_numb)

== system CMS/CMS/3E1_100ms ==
  GaCDP_CellTemp_C : Inport
  GaCDP_BusbarTemp_C : Inport  Port=2
  GcUDS_CellTempNumb_numb : Inport  Port=3
  GcUDS_BusbarTempNumb_numb : Inport  Port=4
  CMS_3E1_100ms : TriggerPort  TriggerType=function-call  VariantControl=(inherit)
  3E1_100ms_sys : Subsystem
  GcCMS_CellTempCnt_numb : Outport
  GcCMS_CellTemp1_C : Outport  Port=2
  GcCMS_CellTemp2_C : Outport  Port=3
  GcCMS_CellTemp3_C : Outport  Port=4
  GcCMS_CellTemp4_C : Outport  Port=5
  GcCMS_CellTemp5_C : Outport  Port=6
  GcCMS_CellTemp6_C : Outport  Port=7
  GcCMS_CellTemp7_C : Outport  Port=8
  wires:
  GaCDP_CellTemp_C/1 -> 3E1_100ms_sys/1(GaCDP_CellTemp_C)
  3E1_100ms_sys/8(GcCMS_CellTemp7_C) -> GcCMS_CellTemp7_C/1
  3E1_100ms_sys/1(GcCMS_CellTempCnt_numb) -> GcCMS_CellTempCnt_numb/1
  3E1_100ms_sys/2(GcCMS_CellTemp1_C) -> GcCMS_CellTemp1_C/1
  3E1_100ms_sys/3(GcCMS_CellTemp2_C) -> GcCMS_CellTemp2_C/1
  3E1_100ms_sys/4(GcCMS_CellTemp3_C) -> GcCMS_CellTemp3_C/1
  3E1_100ms_sys/5(GcCMS_CellTemp4_C) -> GcCMS_CellTemp4_C/1
  3E1_100ms_sys/6(GcCMS_CellTemp5_C) -> GcCMS_CellTemp5_C/1
  3E1_100ms_sys/7(GcCMS_CellTemp6_C) -> GcCMS_CellTemp6_C/1
  GaCDP_BusbarTemp_C/1 -> 3E1_100ms_sys/2(GaCDP_BusbarTemp_C)
  GcUDS_CellTempNumb_numb/1 -> 3E1_100ms_sys/3(GcUDS_CellTempNumb_numb)
  GcUDS_BusbarTempNumb_numb/1 -> 3E1_100ms_sys/4(GcUDS_BusbarTempNumb_numb)

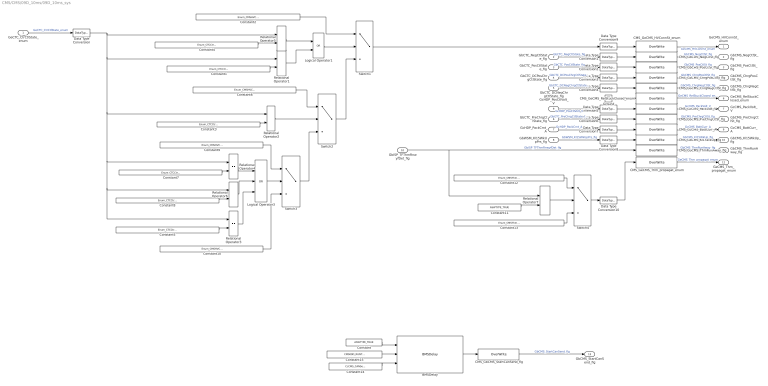
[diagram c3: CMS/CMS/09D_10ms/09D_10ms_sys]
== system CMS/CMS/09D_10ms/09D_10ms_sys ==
  GeCTC_CtrCtlState_enum : Inport
  GbCTC_NegCtlState_flg : Inport  Port=2
  GbCTC_PosCtlState_flg : Inport  Port=3
  GbCTC_DCPosChrgCtlState_flg : Inport  Port=4
  GbCTC_DCNegChrgCtlState_flg : Inport  Port=5
  GbCTC_PreChrgCtlState_flg : Inport  Port=6
  GcHDP_PackCrnt_A : Inport  Port=7
  GbWSM_Kl15WkUpPrs_flg : Inport  Port=8
  GcHDP_PosCtlVolt_V : Inport  Port=9
  GbISP_TFThmRnwyfDet_flg : Inport  Port=10
  BMSDelay : AIWAYS_Powertrain_BMS_lib/Debounce & Delay/BMSDelay
  CMS_GbCMS_ChrgNegCtlSt_flg : AIWAYS_Powertrain_BMS_lib/Signals/OverWrite  OverWrite_Value=CbCMS_ChrgNegCtlStOvr_flg  OverWrite_flag=CbCMS_ChrgNegCtlStOvrSwt_flg
  CMS_GbCMS_ChrgPosCtlSt_flg : AIWAYS_Powertrain_BMS_lib/Signals/OverWrite  OverWrite_Value=CbCMS_ChrgPosCtlStOvr_flg  OverWrite_flag=CbCMS_ChrgPosCtlStOvrSwt_flg
  CMS_GbCMS_Kl15WkUp_flg : AIWAYS_Powertrain_BMS_lib/Signals/OverWrite  OverWrite_Value=CbCMS_Kl15WkUpOvr_flg  OverWrite_flag=CbCMS_Kl15WkUpOvrSwt_flg
  CMS_GbCMS_NegCtlSt_flg : AIWAYS_Powertrain_BMS_lib/Signals/OverWrite  OverWrite_Value=CbCMS_NegCtlStOvr_flg  OverWrite_flag=CbCMS_NegCtlStOvrSwt_flg
  CMS_GbCMS_PosCtlSt_flg : AIWAYS_Powertrain_BMS_lib/Signals/OverWrite  OverWrite_Value=CbCMS_PosCtlStOvr_flg  OverWrite_flag=CbCMS_PosCtlStOvrSwt_flg
  CMS_GbCMS_PreChrgCtlSt_flg : AIWAYS_Powertrain_BMS_lib/Signals/OverWrite  OverWrite_Value=CbCMS_PreChrgCtlStOvr_flg  OverWrite_flag=CbCMS_PreChrgCtlStOvrSwt_flg
  CMS_GbCMS_StartCanSend_flg : AIWAYS_Powertrain_BMS_lib/Signals/OverWrite  OverWrite_Value=CbCMS_StartCanSendOvr_flg  OverWrite_flag=CbCMS_StartCanSendOvrSwt_flg
  CMS_GbCMS_ThmRunAway_flg : AIWAYS_Powertrain_BMS_lib/Signals/OverWrite  OverWrite_Value=CbCMS_ThmRunAwayOvr_flg  OverWrite_flag=CbCMS_ThmRunAwayOvrSwt_flg
  CMS_GcCMS_BattCurr_A : AIWAYS_Powertrain_BMS_lib/Signals/OverWrite  OverWrite_Value=CcCMS_BattCurrOvr_A  OverWrite_flag=CbCMS_BattCurrOvrSwt_flg
  CMS_GcCMS_PackVolt_V : AIWAYS_Powertrain_BMS_lib/Signals/OverWrite  OverWrite_Value=CcCMS_PackVoltOvr_V  OverWrite_flag=CbCMS_PackVoltOvrSwt_flg
  CMS_GeCMS_HVConnSt_enum : AIWAYS_Powertrain_BMS_lib/Signals/OverWrite  OverWrite_Value=CeCMS_HVConnStOvr_enum  OverWrite_flag=CbCMS_HVConnStOvrSwt_flg
  CMS_GeCMS_RelStuckClosed_enum : AIWAYS_Powertrain_BMS_lib/Signals/OverWrite  OverWrite_Value=CeCMS_RelStuckClosedOvr_enum  OverWrite_flag=CbCMS_RelStuckClosedOvrSwt_flg
  CMS_GeCMS_Thm_propagat_enum : AIWAYS_Powertrain_BMS_lib/Signals/OverWrite  OverWrite_Value=CeCMS_ThmOvr_propagat_enum  OverWrite_flag=CbCMS_ThmOvrSwt_flg
  Constant : Constant  Value=ASWTYPE_TRUE
  Constant1 : Constant  Value=Enum_CTCCtrCtlState.Enum_CTCCtrCtlState_Shutdown
  Constant10 : Constant  Value=Enum_CMSHVConnSt.Enum_CMSHVConnSt_Unknown
  Constant11 : Constant  Value=ASWTYPE_TRUE
  Constant12 : Constant  Value=Enum_CMSThmPropagation.Enum_CMSThmPropagation_Runaway
  Constant13 : Constant  Value=Enum_CMSThmPropagation.Enum_CMSThmPropagation_Default
  Constant14 : Constant  Value=CcCMS_CANSendDelay_ms
  Constant15 : Constant  Value=CMS09D_RUNTIME_MS
  Constant2 : Constant  Value=Enum_CMSHVConnSt.Enum_CMSHVConnSt_Disconnect
  Constant3 : Constant  Value=Enum_CTCCtrCtlState.Enum_CTCCtrCtlState_Connect
  Constant4 : Constant  Value=Enum_CTCCtrCtlState.Enum_CTCCtrCtlState_Offline
  Constant5 : Constant  Value=Enum_CTCCtrCtlState.Enum_CTCCtrCtlState_DCConnect
  Constant6 : Constant  Value=Enum_CMSHVConnSt.Enum_CMSHVConnSt_Connecting
  Constant7 : Constant  Value=Enum_CTCCtrCtlState.Enum_CTCCtrCtlState_Online
  Constant8 : Constant  Value=Enum_CTCCtrCtlState.Enum_CTCCtrCtlState_PreShutdown
  Constant9 : Constant  Value=Enum_CMSHVConnSt.Enum_CMSHVConnSt_Connenct
  Data Type Conversion{,1..10} (11 alike) : DataTypeConversion
  Ground : Ground
  Logical Operator1 : Logic  Operator=OR  AllPortsSameDT=off  OutDataTypeStr=boolean
  Logical Operator3 : Logic  Operator=OR  Inputs=3  AllPortsSameDT=off  OutDataTypeStr=boolean
  Relational Operator{1..7} (7 alike) : RelationalOperator  Operator===  OutDataTypeStr=boolean
  Switch{1..4} (4 alike) : Switch  Criteria=u2 ~= 0  Threshold=1  RndMeth=Zero
  GeCMS_HVConnSt_enum : Outport
  GbCMS_NegCtlSt_flg : Outport  Port=2
  GbCMS_PosCtlSt_flg : Outport  Port=3
  GbCMS_ChrgPosCtlSt_flg : Outport  Port=4
  GbCMS_ChrgNegCtlSt_flg : Outport  Port=5
  GeCMS_RelStuckClosed_enum : Outport  Port=6
  GcCMS_PackVolt_V : Outport  Port=7
  GbCMS_PreChrgCtlSt_flg : Outport  Port=8
  GcCMS_BattCurr_A : Outport  Port=9
  GbCMS_Kl15WkUp_flg : Outport  Port=10
  GbCMS_ThmRunAway_flg : Outport  Port=11
  GeCMS_Thm_propagat_enum : Outport  Port=12
  GbCMS_StartCanSend_flg : Outport  Port=13
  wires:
  GeCTC_CtrCtlState_enum/1 -> Data Type Conversion/1  "GeCTC_CtrCtlState_enum"
  CMS_GeCMS_HVConnSt_enum/1 -> GeCMS_HVConnSt_enum/1  "GeCMS_HVConnSt_enum"
  CMS_GbCMS_NegCtlSt_flg/1 -> GbCMS_NegCtlSt_flg/1  "GbCMS_NegCtlSt_flg"
  Data Type Conversion1/1 -> CMS_GbCMS_NegCtlSt_flg/1
  GbCTC_NegCtlState_flg/1 -> Data Type Conversion1/1  "GbCTC_NegCtlState_flg"
  CMS_GbCMS_PosCtlSt_flg/1 -> GbCMS_PosCtlSt_flg/1  "GbCMS_PosCtlSt_flg"
  GbCTC_PosCtlState_flg/1 -> Data Type Conversion2/1  "GbCTC_PosCtlState_flg"
  Data Type Conversion2/1 -> CMS_GbCMS_PosCtlSt_flg/1
  CMS_GbCMS_ChrgPosCtlSt_flg/1 -> GbCMS_ChrgPosCtlSt_flg/1  "GbCMS_ChrgPosCtlSt_flg"
  GbCTC_DCPosChrgCtlState_flg/1 -> Data Type Conversion3/1  "GbCTC_DCPosChrgCtlState_flg"
  Data Type Conversion3/1 -> CMS_GbCMS_ChrgPosCtlSt_flg/1
  CMS_GbCMS_ChrgNegCtlSt_flg/1 -> GbCMS_ChrgNegCtlSt_flg/1  "GbCMS_ChrgNegCtlSt_flg"
  GbCTC_DCNegChrgCtlState_flg/1 -> Data Type Conversion4/1  "GbCTC_DCNegChrgCtlState_flg"
  Data Type Conversion4/1 -> CMS_GbCMS_ChrgNegCtlSt_flg/1
  CMS_GeCMS_RelStuckClosed_enum/1 -> GeCMS_RelStuckClosed_enum/1  "GeCMS_RelStuckClosed_enum"
  Ground/1 -> CMS_GeCMS_RelStuckClosed_enum/1
  GcHDP_PosCtlVolt_V/1 -> Data Type Conversion5/1  "GcHDP_PosCtlVolt_V"
  Data Type Conversion5/1 -> CMS_GcCMS_PackVolt_V/1
  GbCTC_PreChrgCtlState_flg/1 -> Data Type Conversion6/1  "GbCTC_PreChrgCtlState_flg"
  Data Type Conversion6/1 -> CMS_GbCMS_PreChrgCtlSt_flg/1
  CMS_GcCMS_BattCurr_A/1 -> GcCMS_BattCurr_A/1  "GcCMS_BattCurr_A"
  Data Type Conversion7/1 -> CMS_GcCMS_BattCurr_A/1
  GcHDP_PackCrnt_A/1 -> Data Type Conversion7/1  "GcHDP_PackCrnt_A"
  CMS_GbCMS_Kl15WkUp_flg/1 -> GbCMS_Kl15WkUp_flg/1  "GbCMS_Kl15WkUp_flg"
  GbWSM_Kl15WkUpPrs_flg/1 -> Data Type Conversion8/1  "GbWSM_Kl15WkUpPrs_flg"
  Data Type Conversion8/1 -> CMS_GbCMS_Kl15WkUp_flg/1
  CMS_GbCMS_ThmRunAway_flg/1 -> GbCMS_ThmRunAway_flg/1  "GbCMS_ThmRunAway_flg"
  CMS_GcCMS_PackVolt_V/1 -> GcCMS_PackVolt_V/1  "GcCMS_PackVolt_V"
  CMS_GbCMS_PreChrgCtlSt_flg/1 -> GbCMS_PreChrgCtlSt_flg/1  "GbCMS_PreChrgCtlSt_flg"
  Constant4/1 -> Relational Operator5/2
  Relational Operator5/1 -> Logical Operator1/1
  Constant2/1 -> Switch1/1
  Constant3/1 -> Relational Operator2/2
  Constant5/1 -> Relational Operator3/2
  Relational Operator3/1 -> Logical Operator3/3
  Relational Operator2/1 -> Switch2/2
  Switch2/1 -> Switch1/3
  Constant6/1 -> Switch2/1
  Relational Operator6/1 -> Logical Operator3/2
  Relational Operator4/1 -> Logical Operator3/1
  Constant8/1 -> Relational Operator6/2
  Constant7/1 -> Relational Operator4/2
  Logical Operator3/1 -> Switch3/2
  Constant9/1 -> Switch3/1
  Constant10/1 -> Switch3/3
  Switch3/1 -> Switch2/3
  Switch1/1 -> Data Type Conversion9/1
  Data Type Conversion9/1 -> CMS_GeCMS_HVConnSt_enum/1
  Switch4/1 -> Data Type Conversion10/1
  CMS_GeCMS_Thm_propagat_enum/1 -> GeCMS_Thm_propagat_enum/1  "GeCMS_Thm_propagat_enum"
  Constant1/1 -> Relational Operator1/2
  Data Type Conversion/1 -> Relational Operator1/1, Relational Operator2/1, Relational Operator4/1, Relational Operator6/1, Relational Operator3/1, Relational Operator5/1
  Relational Operator1/1 -> Logical Operator1/2
  Constant11/1 -> Relational Operator7/2
  GbISP_TFThmRnwyfDet_flg/1 -> Relational Operator7/1, CMS_GbCMS_ThmRunAway_flg/1  "GbISP_TFThmRnwyfDet_flg"
  Relational Operator7/1 -> Switch4/2
  Constant12/1 -> Switch4/1
  Constant13/1 -> Switch4/3
  Data Type Conversion10/1 -> CMS_GeCMS_Thm_propagat_enum/1
  Constant14/1 -> BMSDelay/3
  Constant15/1 -> BMSDelay/2
  Constant/1 -> BMSDelay/1
  BMSDelay/1 -> CMS_GbCMS_StartCanSend_flg/1
  CMS_GbCMS_StartCanSend_flg/1 -> GbCMS_StartCanSend_flg/1  "GbCMS_StartCanSend_flg"
  Logical Operator1/1 -> Switch1/2

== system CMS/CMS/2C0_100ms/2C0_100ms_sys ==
  GcLDP_lntWtTemp_C : Inport
  GcLDP_OutWtTemp_C : Inport  Port=2
  GcBTM_CoolPwrReq_W : Inport  Port=3
  GcBTM_HeatPwrReq_W : Inport  Port=4
  GeBTM_CoolReq_enum : Inport  Port=5
  GeBTM_HeatReq_enum : Inport  Port=6
  CMS_GcCMS_CoolPwrReq_W : AIWAYS_Powertrain_BMS_lib/Signals/OverWrite  OverWrite_Value=CcCMS_CoolPwrReqOvr_W  OverWrite_flag=CbCMS_CoolPwrReqOvrSwt_flg
  CMS_GcCMS_CoolTempIn_C : AIWAYS_Powertrain_BMS_lib/Signals/OverWrite  OverWrite_Value=CcCMS_CoolTempInOvr_C  OverWrite_flag=CbCMS_CoolTempInOvrSwt_flg
  CMS_GcCMS_CoolTempOut_C : AIWAYS_Powertrain_BMS_lib/Signals/OverWrite  OverWrite_Value=CcCMS_CoolTempOutOvr_C  OverWrite_flag=CbCMS_CoolTempOutOvrSwt_flg
  CMS_GcCMS_HeatPwrReq_W : AIWAYS_Powertrain_BMS_lib/Signals/OverWrite  OverWrite_Value=CcCMS_HeatPwrReqOvr_W  OverWrite_flag=CbCMS_HeatPwrReqOvrSwt_flg
  CMS_GeCMS_CoolReq_enum : AIWAYS_Powertrain_BMS_lib/Signals/OverWrite  OverWrite_Value=CeCMS_CoolReqOvr_enum  OverWrite_flag=CbCMS_CoolReqOvrSwt_flg
  CMS_GeCMS_HeatReq_enum : AIWAYS_Powertrain_BMS_lib/Signals/OverWrite  OverWrite_Value=CeCMS_HeatReqOvr_enum  OverWrite_flag=CbCMS_HeatReqOvrSwt_flg
  Data Type Conversion{2..7} (6 alike) : DataTypeConversion
  GcCMS_CoolTempIn_C : Outport
  GcCMS_CoolTempOut_C : Outport  Port=2
  GcCMS_CoolPwrReq_W : Outport  Port=3
  GcCMS_HeatPwrReq_W : Outport  Port=4
  GeCMS_CoolReq_enum : Outport  Port=5
  GeCMS_HeatReq_enum : Outport  Port=6
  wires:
  CMS_GcCMS_CoolTempIn_C/1 -> GcCMS_CoolTempIn_C/1  "GcCMS_CoolTempIn_C"
  CMS_GcCMS_CoolTempOut_C/1 -> GcCMS_CoolTempOut_C/1  "GcCMS_CoolTempOut_C"
  CMS_GeCMS_HeatReq_enum/1 -> GeCMS_HeatReq_enum/1  "GeCMS_HeatReq_enum"
  CMS_GeCMS_CoolReq_enum/1 -> GeCMS_CoolReq_enum/1  "GeCMS_CoolReq_enum"
  CMS_GcCMS_HeatPwrReq_W/1 -> GcCMS_HeatPwrReq_W/1  "GcCMS_HeatPwrReq_W"
  CMS_GcCMS_CoolPwrReq_W/1 -> GcCMS_CoolPwrReq_W/1  "GcCMS_CoolPwrReq_W"
  GcLDP_lntWtTemp_C/1 -> Data Type Conversion4/1
  GcLDP_OutWtTemp_C/1 -> Data Type Conversion5/1
  GcBTM_CoolPwrReq_W/1 -> Data Type Conversion6/1
  GcBTM_HeatPwrReq_W/1 -> Data Type Conversion7/1
  GeBTM_CoolReq_enum/1 -> Data Type Conversion3/1
  GeBTM_HeatReq_enum/1 -> Data Type Conversion2/1
  Data Type Conversion2/1 -> CMS_GeCMS_HeatReq_enum/1
  Data Type Conversion3/1 -> CMS_GeCMS_CoolReq_enum/1
  Data Type Conversion4/1 -> CMS_GcCMS_CoolTempIn_C/1
  Data Type Conversion5/1 -> CMS_GcCMS_CoolTempOut_C/1
  Data Type Conversion6/1 -> CMS_GcCMS_CoolPwrReq_W/1
  Data Type Conversion7/1 -> CMS_GcCMS_HeatPwrReq_W/1

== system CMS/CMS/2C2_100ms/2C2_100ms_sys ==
  GcSOP_DischrgPwr_kW : Inport
  GcSOP_ChrgPwr_kW : Inport  Port=2
  GcHDP_PackVolt_V : Inport  Port=3
  CMS_GcCMS_PeakCurrCh_A : AIWAYS_Powertrain_BMS_lib/Signals/OverWrite  OverWrite_Value=CcCMS_PeakCurrChOvr_A  OverWrite_flag=CbCMS_PeakCurrChOvrSwt_flg
  CMS_GcCMS_PeakCurrDisCh_A : AIWAYS_Powertrain_BMS_lib/Signals/OverWrite  OverWrite_Value=CcCMS_PeakCurrDisChOvr_A  OverWrite_flag=CbCMS_PeakCurrDisChOvrSwt_flg
  CMS_GcCMS_PeakVoltCh_V : AIWAYS_Powertrain_BMS_lib/Signals/OverWrite  OverWrite_Value=CcCMS_PeakVoltChOvr_V  OverWrite_flag=CbCMS_PeakVoltChOvrSwt_flg
  CMS_GcCMS_PeakVoltDisCh_V : AIWAYS_Powertrain_BMS_lib/Signals/OverWrite  OverWrite_Value=CcCMS_PeakVoltDisChOvr_V  OverWrite_flag=CbCMS_PeakVoltDisChOvrSwt_flg
  Constant1 : Constant  Value=CMS_CONST1000_NUMB
  Constant14 : Constant  Value=CMS_CONST1000_NUMB
  Constant2 : Constant  Value=CcCMS_PeakVoltDisCh_V
  Constant3 : Constant  Value=CcCMS_PeakVoltCh_V
  Constant5 : Constant  Value=CMS_CONSTF1_NUMB
  Data Type Conversion : DataTypeConversion
  Data Type Conversion1 : DataTypeConversion
  Product : Product  OutDataTypeStr=Inherit: Inherit via back propagation
  Product1 : Product  Inputs=*/  OutDataTypeStr=Inherit: Inherit via back propagation
  Product2 : Product  OutDataTypeStr=Inherit: Inherit via back propagation
  Product3 : Product  Inputs=*/  OutDataTypeStr=Inherit: Inherit via back propagation
  Product4 : Product  OutDataTypeStr=Inherit: Inherit via back propagation
  GcCMS_PeakCurrDisCh_A : Outport
  GcCMS_PeakCurrCh_A : Outport  Port=2
  GcCMS_PeakVoltDisCh_V : Outport  Port=3
  GcCMS_PeakVoltCh_V : Outport  Port=4
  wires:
  CMS_GcCMS_PeakCurrDisCh_A/1 -> GcCMS_PeakCurrDisCh_A/1  "GcCMS_PeakCurrDisCh_A"
  CMS_GcCMS_PeakCurrCh_A/1 -> GcCMS_PeakCurrCh_A/1  "GcCMS_PeakCurrCh_A"
  CMS_GcCMS_PeakVoltDisCh_V/1 -> GcCMS_PeakVoltDisCh_V/1  "GcCMS_PeakVoltDisCh_V"
  CMS_GcCMS_PeakVoltCh_V/1 -> GcCMS_PeakVoltCh_V/1  "GcCMS_PeakVoltCh_V"
  Data Type Conversion/1 -> CMS_GcCMS_PeakCurrDisCh_A/1
  Data Type Conversion1/1 -> CMS_GcCMS_PeakCurrCh_A/1
  Constant2/1 -> CMS_GcCMS_PeakVoltDisCh_V/1
  Constant3/1 -> CMS_GcCMS_PeakVoltCh_V/1
  GcSOP_DischrgPwr_kW/1 -> Product/1  "GcSOP_DischrgPwr_kW"
  GcSOP_ChrgPwr_kW/1 -> Product2/1  "GcSOP_ChrgPwr_kW"
  GcHDP_PackVolt_V/1 -> Product3/2, Product1/2  "GcHDP_PackVolt_V"
  Product1/1 -> Data Type Conversion/1
  Constant14/1 -> Product/2
  Product/1 -> Product1/1
  Product2/1 -> Product3/1
  Constant1/1 -> Product2/2
  Product3/1 -> Product4/1
  Constant5/1 -> Product4/2
  Product4/1 -> Data Type Conversion1/1

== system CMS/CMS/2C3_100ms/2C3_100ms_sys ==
  GcCDP_MinCellVolt_mV : Inport
  GcCDP_MaxCellVolt_mV : Inport  Port=2
  GcBTM_CoolTempReq_C : Inport  Port=3
  GcBTM_HeatTempReq_C : Inport  Port=4
  GcCDP_MaxBusbarTemp_C : Inport  Port=5
  GcCDP_MinBusbarTemp_C : Inport  Port=6
  GcUDS_BusbarTempNumb_numb : Inport  Port=7
  GcCDP_MaxCellTemp_C : Inport  Port=8
  GcCDP_MinCellTemp_C : Inport  Port=9
  CMS_GcCMS_BusbarTempMax_C : AIWAYS_Powertrain_BMS_lib/Signals/OverWrite  OverWrite_Value=CcCMS_BusbarTempMaxOvr_C  OverWrite_flag=CbCMS_BusbarTempMaxOvrSwt_flg
  CMS_GcCMS_BusbarTempMin_C : AIWAYS_Powertrain_BMS_lib/Signals/OverWrite  OverWrite_Value=CcCMS_BusbarTempMinOvr_C  OverWrite_flag=CbCMS_BusbarTempMinOvrSwt_flg
  CMS_GcCMS_ClntTgtTemp_C : AIWAYS_Powertrain_BMS_lib/Signals/OverWrite  OverWrite_Value=CcCMS_ClntTgtTempOvr_C  OverWrite_flag=CbCMS_ClntTgtTempOvrSwt_flg
  CMS_GcCMS_HtTgtTemp_C : AIWAYS_Powertrain_BMS_lib/Signals/OverWrite  OverWrite_Value=CcCMS_HtTgtTempOvr_C  OverWrite_flag=CbCMS_HtTgtTempOvrSwt_flg
  CMS_GcCMS_MaxCellVolt_V : AIWAYS_Powertrain_BMS_lib/Signals/OverWrite  OverWrite_Value=CcCMS_MaxCellVoltOvr_V  OverWrite_flag=CbCMS_MaxCellVoltOvrSwt_flg
  CMS_GcCMS_MinCellVolt_V : AIWAYS_Powertrain_BMS_lib/Signals/OverWrite  OverWrite_Value=CcCMS_MinCellVoltOvr_V  OverWrite_flag=CbCMS_MinCellVoltOvrSwt_flg
  Constant1 : Constant  Value=CMS_CONST1000_NUMB
  Constant2 : Constant  Value=CMS_CONST1000_NUMB
  Constant3 : Constant  Value=CMS_CONST0_NUMB
  Data Type Conversion{,1,4..5} (4 alike) : DataTypeConversion  RndMeth=Round
  Data Type Conversion2 : DataTypeConversion
  Data Type Conversion3 : DataTypeConversion
  Product1 : Product  Inputs=*/  OutDataTypeStr=single
  Product2 : Product  Inputs=*/  OutDataTypeStr=single
  Relational Operator1 : RelationalOperator  Operator=>  OutDataTypeStr=boolean
  Switch1 : Switch  Criteria=u2 ~= 0  Threshold=1  RndMeth=Zero
  Switch2 : Switch  Criteria=u2 ~= 0  Threshold=1  RndMeth=Zero
  GcCMS_ClntTgtTemp_C : Outport
  GcCMS_HtTgtTemp_C : Outport  Port=2
  GcCMS_MaxCellVolt_V : Outport  Port=3
  GcCMS_BusbarTempMax_C : Outport  Port=4
  GcCMS_BusbarTempMin_C : Outport  Port=5
  GcCMS_MinCellVolt_V : Outport  Port=6
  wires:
  CMS_GcCMS_ClntTgtTemp_C/1 -> GcCMS_ClntTgtTemp_C/1  "GcCMS_ClntTgtTemp_C"
  CMS_GcCMS_BusbarTempMin_C/1 -> GcCMS_BusbarTempMin_C/1  "GcCMS_BusbarTempMin_C"
  CMS_GcCMS_BusbarTempMax_C/1 -> GcCMS_BusbarTempMax_C/1  "GcCMS_BusbarTempMax_C"
  CMS_GcCMS_MaxCellVolt_V/1 -> GcCMS_MaxCellVolt_V/1  "GcCMS_MaxCellVolt_V"
  CMS_GcCMS_HtTgtTemp_C/1 -> GcCMS_HtTgtTemp_C/1  "GcCMS_HtTgtTemp_C"
  Constant2/1 -> Product1/2
  GcCDP_MinCellVolt_mV/1 -> Product1/1  "GcCDP_MinCellVolt_mV"
  CMS_GcCMS_MinCellVolt_V/1 -> GcCMS_MinCellVolt_V/1  "GcCMS_MinCellVolt_V"
  Product1/1 -> Data Type Conversion/1
  GcBTM_CoolTempReq_C/1 -> Data Type Conversion2/1  "GcBTM_CoolTempReq_C"
  GcBTM_HeatTempReq_C/1 -> Data Type Conversion3/1  "GcBTM_HeatTempReq_C"
  GcCDP_MaxBusbarTemp_C/1 -> Switch1/1  "GcCDP_MaxBusbarTemp_C"
  GcCDP_MinBusbarTemp_C/1 -> Switch2/1  "GcCDP_MinBusbarTemp_C"
  Data Type Conversion/1 -> CMS_GcCMS_MinCellVolt_V/1
  GcCDP_MaxCellVolt_mV/1 -> Product2/1  "GcCDP_MaxCellVolt_mV"
  Product2/1 -> Data Type Conversion1/1
  Constant1/1 -> Product2/2
  Data Type Conversion1/1 -> CMS_GcCMS_MaxCellVolt_V/1
  Data Type Conversion2/1 -> CMS_GcCMS_ClntTgtTemp_C/1
  Data Type Conversion3/1 -> CMS_GcCMS_HtTgtTemp_C/1
  Data Type Conversion4/1 -> CMS_GcCMS_BusbarTempMax_C/1
  Data Type Conversion5/1 -> CMS_GcCMS_BusbarTempMin_C/1
  GcUDS_BusbarTempNumb_numb/1 -> Relational Operator1/1
  Constant3/1 -> Relational Operator1/2
  Relational Operator1/1 -> Switch2/2, Switch1/2
  GcCDP_MaxCellTemp_C/1 -> Switch1/3
  Switch1/1 -> Data Type Conversion4/1
  GcCDP_MinCellTemp_C/1 -> Switch2/3
  Switch2/1 -> Data Type Conversion5/1
